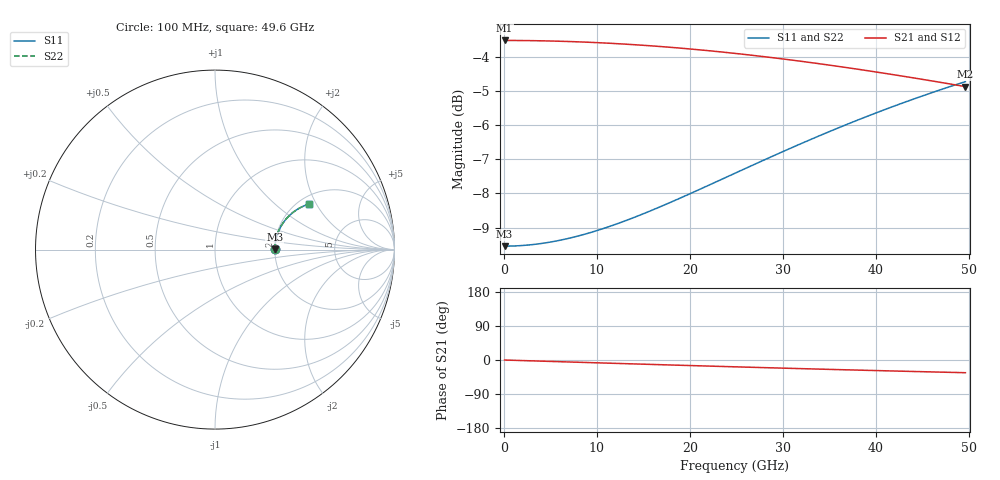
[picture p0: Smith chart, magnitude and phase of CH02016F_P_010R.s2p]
# GHz S RI R 10
! S-Parameters data
! Freq  reS11  imS11  reS21  imS21  reS12  imS12  reS22  imS22
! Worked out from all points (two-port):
!   100 points, 100 MHz to 49.6 GHz, reference 10 ohm
!   highest |S21| = -3.52 dB at 100 MHz (marker M1); lowest = -4.9 dB at 49.6 GHz (marker M2)
!   |S21| within 3 dB of the highest: start of sweep to end of sweep
!   lowest |S11| = -9.5 dB at 100 MHz (marker M3), VSWR 2.00, Z = 20 + j0.0333 ohm
!   |S11| at or under -10 dB: nowhere
!   |S22| runs from -9.5 to -4.7 dB; largest |S21 - S12| = 0
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0.1  0.3333 0.00074  0.6667 -0.000866  0.6667 -0.000866  0.3333 0.00074
2.1  0.3338 0.0155  0.6662 -0.0182  0.6662 -0.0182  0.3338 0.0155
4.1  0.3351 0.0303  0.6649 -0.0354  0.6649 -0.0354  0.3351 0.0303
6.1  0.3372 0.0449  0.6628 -0.0525  0.6628 -0.0525  0.3372 0.0449
8.6  0.341 0.0628  0.659 -0.0736  0.659 -0.0736  0.341 0.0628
10.1  0.3438 0.0735  0.6561 -0.0861  0.6561 -0.0861  0.3438 0.0735
12.1  0.3483 0.0873  0.6516 -0.1025  0.6516 -0.1025  0.3483 0.0873
14.1  0.3535 0.1009  0.6463 -0.1186  0.6463 -0.1186  0.3535 0.1009
16.6  0.361 0.1173  0.6388 -0.1381  0.6388 -0.1381  0.361 0.1173
18.6  0.3678 0.1299  0.632 -0.1532  0.632 -0.1532  0.3678 0.1299
20.6  0.3751 0.142  0.6246 -0.1679  0.6246 -0.1679  0.3751 0.142
23.1  0.3851 0.1564  0.6145 -0.1854  0.6145 -0.1854  0.3851 0.1564
25.1  0.3936 0.1674  0.6059 -0.1989  0.6059 -0.1989  0.3936 0.1674
29.1  0.4121 0.1875  0.5872 -0.224  0.5872 -0.224  0.4121 0.1875
31.1  0.4219 0.1967  0.5773 -0.2357  0.5773 -0.2357  0.4219 0.1967
33.1  0.432 0.2052  0.5671 -0.2468  0.5671 -0.2468  0.432 0.2052
35.1  0.4424 0.2132  0.5566 -0.2573  0.5566 -0.2573  0.4424 0.2132
37.1  0.4531 0.2205  0.5458 -0.2671  0.5458 -0.2671  0.4531 0.2205
39.1  0.4639 0.2272  0.5349 -0.2763  0.5349 -0.2763  0.4639 0.2272
41.6  0.4776 0.2348  0.521 -0.287  0.521 -0.287  0.4776 0.2348
45.6  0.4999 0.2449  0.4985 -0.3022  0.4985 -0.3022  0.4999 0.2449
49.6  0.5223 0.2528  0.4758 -0.3151  0.4758 -0.3151  0.5223 0.2528
